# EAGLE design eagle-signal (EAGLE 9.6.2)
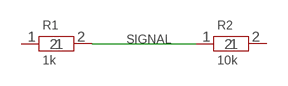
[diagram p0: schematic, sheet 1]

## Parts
R1  1k  R  [R0603]
R2  10k  R  [R0603]

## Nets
SIGNAL: R1.2 R2.1
Unconnected: R1.1 R2.2

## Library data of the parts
R1 R2 = maker:R

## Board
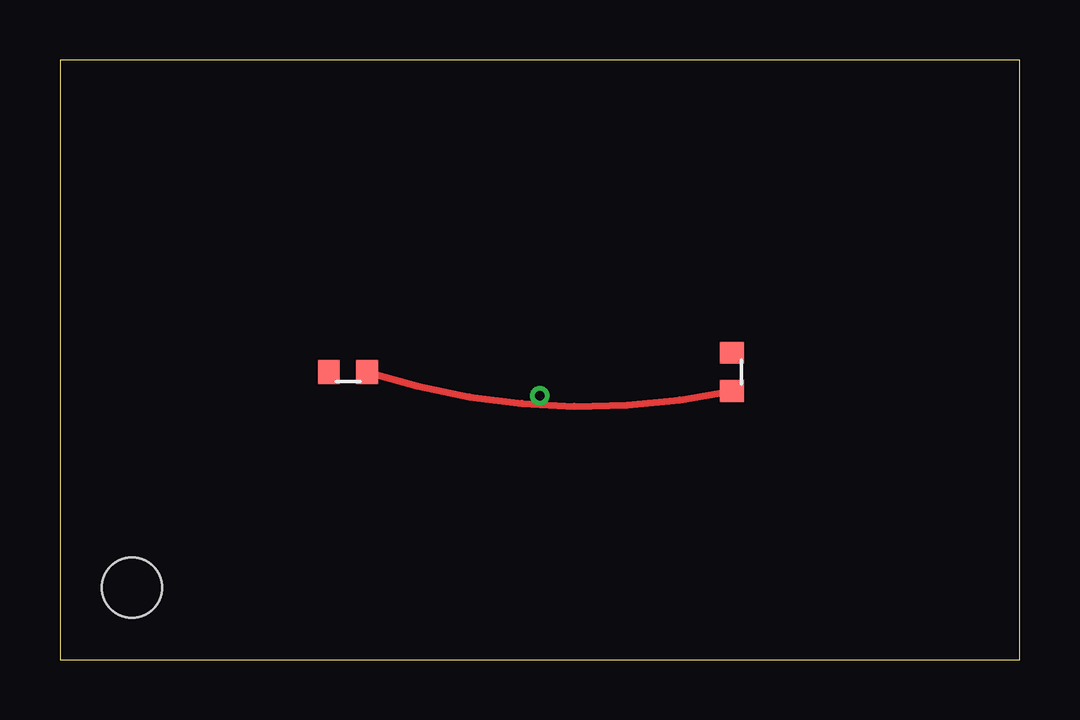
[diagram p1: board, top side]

Size 40 x 25 mm. Coordinates in mm from the lower left corner, seen from the top.
Outline: 0,0 40,0 40,25 0,25 0,0
Copper layers used: Top
Holes 2.5 mm at 3,3

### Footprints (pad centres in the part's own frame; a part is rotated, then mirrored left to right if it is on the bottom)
R0603 = smd 0.9 x 1: 1 -0.8,0; 2 0.8,0

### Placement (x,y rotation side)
R1  12,12 0 top
R2  28,12 90 top

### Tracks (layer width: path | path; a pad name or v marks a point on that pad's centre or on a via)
SIGNAL  (via drill 0.4 pad 0.8)
  Top 0.3: R1.2 arc30 R2.1
  other vias: 20,11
